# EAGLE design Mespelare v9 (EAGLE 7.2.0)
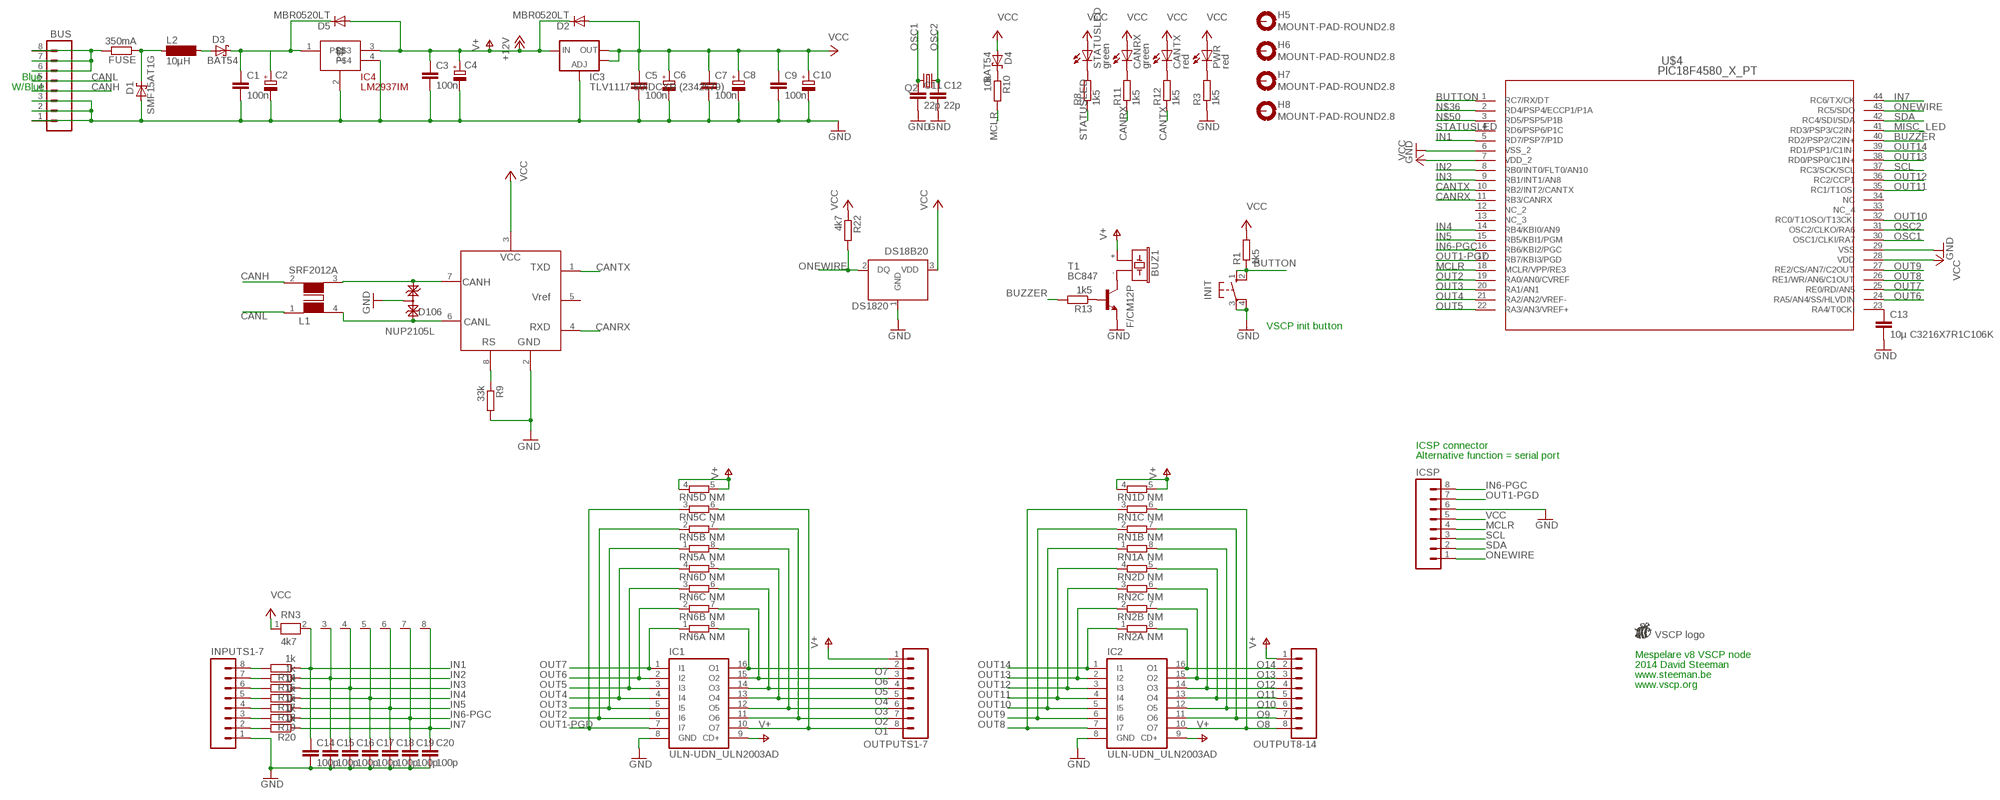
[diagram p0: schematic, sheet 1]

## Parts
BUS  M083.5MM-8  [SCREWTERMINAL-3.5MM-8]
BUZ1  F/CM12P  [F/CM12P]
C1  100n  C-EUC1206K  [C1206K]
C2  CPOL-EUC  [PANASONIC_C]
C3  100n  C-EUC1206K  [C1206K]
C4  CPOL-EUC  [PANASONIC_C]
C5  100n  C-EUC1206K  [C1206K]
C6  CPOL-EUC  [PANASONIC_C]
C7  100n  C-EUC1206K  [C1206K]
C8  CPOL-EUC  [PANASONIC_C]
C9  100n  C-EUC1206K  [C1206K]
C10  CPOL-EUC  [PANASONIC_C]
C11  22p  C-EUC1206  [C1206]
C12  22p  C-EUC1206  [C1206]
C13  10µ C3216X7R1C106K  C-EUC1206K  [C1206K]
C14  100p  C-EUC1206  [C1206]
C15  100p  C-EUC1206  [C1206]
C16  100p  C-EUC1206  [C1206]
C17  100p  C-EUC1206  [C1206]
C18  100p  C-EUC1206  [C1206]
C19  100p  C-EUC1206  [C1206]
C20  100p  C-EUC1206  [C1206]
CANRX  green  LEDCHIPLED_1206  [CHIPLED_1206]
CANTX  red  LEDCHIPLED_1206  [CHIPLED_1206]
D1  SMF15AT1G  SMF5.0AT1  [SOD123FL]
D2  MBR0520LT  [SOD123]
D3  BAT54  [SOT23]
D4  BAT54  [SOT23]
D5  MBR0520LT  [SOD123]
D106  NUP2105L  NUP2105LSOT23  [DIODE_SOT23]
DS18B20  DS1820  [TO-92]
FUSE  350mA  R-EU_M1206  [M1206]
H5  MOUNT-PAD-ROUND2.8  [2,2-PAD2]
H6  MOUNT-PAD-ROUND2.8  [2,2-PAD2]
H7  MOUNT-PAD-ROUND2.8  [2,2-PAD2]
H8  MOUNT-PAD-ROUND2.8  [2,2-PAD2]
IC1  ULN-UDN_ULN2003AD  [ULN-UDN_SO16]
IC2  ULN-UDN_ULN2003AD  [ULN-UDN_SO16]
IC3  TLV1117-50IDCYR (2342579)  LD117ASTR  [SOT223]
IC4  LM2937IM  [SOT223]
ICSP  M083.5MM-8  [SCREWTERMINAL-3.5MM-8]
INIT  10-XX  [B3F-10XX]
INPUTS1-7  M083.5MM-8  [SCREWTERMINAL-3.5MM-8]
L1  SRF2012A  [SRF2012A]
L2  10µH  SM-NE45  [SM-NE45]
OUTPUT8-14  M083.5MM-8  [SCREWTERMINAL-3.5MM-8]
OUTPUTS1-7  M083.5MM-8  [SCREWTERMINAL-3.5MM-8]
PWR  red  LEDCHIPLED_1206  [CHIPLED_1206]
Q2  CRYSTALHC49UP  [HC49UP]
R1  1k5  R-EU_M1206  [M1206]
R3  1k5  R-EU_M1206  [M1206]
R8  1k5  R-EU_M1206  [M1206]
R9  33k  R-EU_M1206  [M1206]
R10  10k  R-EU_M1206  [M1206]
R11  1k5  R-EU_M1206  [M1206]
R12  1k5  R-EU_M1206  [M1206]
R13  1k5  R-EU_M1206  [M1206]
R14  1k  R-EU_M1206  [M1206]
R15  1k  R-EU_M1206  [M1206]
R16  1k  R-EU_M1206  [M1206]
R17  1k  R-EU_M1206  [M1206]
R18  1k  R-EU_M1206  [M1206]
R19  1k  R-EU_M1206  [M1206]
R20  1k  R-EU_M1206  [M1206]
R22  4k7  R-EU_M1206  [M1206]
RN1  NM  4R-NEXBS8V  [EXBS8V]
RN2  NM  4R-NEXBS8V  [EXBS8V]
RN3  4k7  RN07  [RN-8]
RN5  NM  4R-NEXBS8V  [EXBS8V]
RN6  NM  4R-NEXBS8V  [EXBS8V]
STATUSLED  green  LEDCHIPLED_1206  [CHIPLED_1206]
T1  BC847  [SOT23]
U101  MCP2551  [MCP2551]
U$1  VSCP_LOGO2  [VSCP_LOGO2]
U$4  PIC18F4580_X_PT  [TQFP44_MC]

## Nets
BUTTON: INIT.1(S) INIT.2(S1) R1.1 U$4.1(RC7/RX/DT)
BUZZER: R13.2 U$4.40(RD2/PSP2/C2IN+)
CANH: BUS.4 L1.2
CANL: BUS.5 L1.1
CANRX: R11.1 U101.4(RXD) U$4.11(RB3/CANRX)
CANTX: R12.1 U101.1(TXD) U$4.10(RB2/INT2/CANTX)
GND: BUS.1 BUS.2 BUS.3 C1.2 C2.- C3.2 C4.- C5.2 C6.- C7.2 C8.- C9.2 C10.- C11.2 C12.2 C13.2 C14.2 C15.2 C16.2 C17.2 C18.2 C19.2 C20.2 D1.A D106.3(A) DS18B20.1(GND) IC1.8(GND) IC2.8(GND) IC3.1(ADJ) IC4.2 IC4.4 ICSP.6 INIT.3(P) INIT.4(P1) INPUTS1-7.1 R3.1 R9.2 T1.2(E) U101.2(GND) U$4.6(VSS_2) U$4.29(VSS)
I1: INPUTS1-7.8 R14.2
I2: INPUTS1-7.7 R15.2
I3: INPUTS1-7.6 R16.2
I4: INPUTS1-7.5 R17.2
I5: INPUTS1-7.4 R18.2
I6: INPUTS1-7.3 R19.2
I7: INPUTS1-7.2 R20.2
IN1: C14.1 R14.1 RN3.2 U$4.5(RD7/PSP7/P1D)
IN2: C15.1 R15.1 RN3.3 U$4.8(RB0/INT0/FLT0/AN10)
IN3: C16.1 R16.1 RN3.4 U$4.9(RB1/INT1/AN8)
IN4: C17.1 R17.1 RN3.5 U$4.14(RB4/KBI0/AN9)
IN5: C18.1 R18.1 RN3.6 U$4.15(RB5/KBI1/PGM)
IN6-PGC: C19.1 ICSP.8 R19.1 RN3.7 U$4.16(RB6/KBI2/PGC)
IN7: C20.1 R20.1 RN3.8 U$4.44(RC6/TX/CK)
MCLR: ICSP.4 R10.2 U$4.18(MCLR/VPP/RE3)
MISC_LED: U$4.41(RD3/PSP3/C2IN-)
N$1: D106.1(K1) L1.4 U101.6(CANL)
N$2: D106.2(K2) L1.3 U101.7(CANH)
N$3: C13.1 U$4.23(RA4/T0CKI)
N$5: C1.1 C2.+ D3.3(C) D5.C IC4.1
N$6: D1.C FUSE.1 L2.1
N$7: R9.1 U101.8(RS)
N$14: BUS.6 BUS.7 BUS.8 FUSE.2
N$15: D4.3(C) R10.1
N$16: R8.2 STATUSLED.C
N$19: D3.1(A) L2.2
N$20: BUZ1.- T1.3(C)
N$24: PWR.C R3.2
N$27: R13.1 T1.1(B)
N$36: U$4.2(RD4/PSP4/ECCP1/P1A)
N$50: U$4.3(RD5/PSP5/P1B)
N$53: CANRX.C R11.2
N$54: CANTX.C R12.2
O1: IC1.10(O7) OUTPUTS1-7.8 RN5.6
O2: IC1.11(O6) OUTPUTS1-7.7 RN5.7
O3: IC1.12(O5) OUTPUTS1-7.6 RN5.8
O4: IC1.13(O4) OUTPUTS1-7.5 RN6.5
O5: IC1.14(O3) OUTPUTS1-7.4 RN6.6
O6: IC1.15(O2) OUTPUTS1-7.3 RN6.7
O7: IC1.16(O1) OUTPUTS1-7.2 RN6.8
O8: IC2.10(O7) OUTPUT8-14.8 RN1.6
O9: IC2.11(O6) OUTPUT8-14.7 RN1.7
O10: IC2.12(O5) OUTPUT8-14.6 RN1.8
O11: IC2.13(O4) OUTPUT8-14.5 RN2.5
O12: IC2.14(O3) OUTPUT8-14.4 RN2.6
O13: IC2.15(O2) OUTPUT8-14.3 RN2.7
O14: IC2.16(O1) OUTPUT8-14.2 RN2.8
ONEWIRE: DS18B20.2(DQ) ICSP.1 R22.2 U$4.43(RC5/SDO)
OSC1: C11.1 Q2.2 U$4.30(OSC1/CLKI/RA7)
OSC2: C12.1 Q2.1 U$4.31(OSC2/CLKO/RA6)
OUT1-PGD: IC1.7(I7) ICSP.7 RN5.3 U$4.17(RB7/KBI3/PGD)
OUT2: IC1.6(I6) RN5.2 U$4.19(RA0/AN0/CVREF)
OUT3: IC1.5(I5) RN5.1 U$4.20(RA1/AN1)
OUT4: IC1.4(I4) RN6.4 U$4.21(RA2/AN2/VREF-)
OUT5: IC1.3(I3) RN6.3 U$4.22(RA3/AN3/VREF+)
OUT6: IC1.2(I2) RN6.2 U$4.24(RA5/AN4/SS/HLVDIN)
OUT7: IC1.1(I1) RN6.1 U$4.25(RE0/RD/AN5)
OUT8: IC2.7(I7) RN1.3 U$4.26(RE1/WR/AN6/C1OUT)
OUT9: IC2.6(I6) RN1.2 U$4.27(RE2/CS/AN7/C2OUT)
OUT10: IC2.5(I5) RN1.1 U$4.32(RC0/T1OSO/T13CKI)
OUT11: IC2.4(I4) RN2.4 U$4.35(RC1/T1OSI)
OUT12: IC2.3(I3) RN2.3 U$4.36(RC2/CCP1)
OUT13: IC2.2(I2) RN2.2 U$4.38(RD0/PSP0/C1IN+)
OUT14: IC2.1(I1) RN2.1 U$4.39(RD1/PSP1/C1IN-)
SCL: ICSP.3 U$4.37(RC3/SCK/SCL)
SDA: ICSP.2 U$4.42(RC4/SDI/SDA)
STATUSLED: R8.1 U$4.4(RD6/PSP6/P1C)
V+: BUZ1.+ C3.1 C4.+ D2.C D5.A IC1.9(CD+) IC2.9(CD+) IC3.3(IN) IC4.3 OUTPUT8-14.1 OUTPUTS1-7.1 RN1.4 RN1.5 RN5.4 RN5.5 ; supply symbol labelled +12V
VCC: C5.1 C6.+ C7.1 C8.+ C9.1 C10.+ CANRX.A CANTX.A D2.A D4.1(A) DS18B20.3(VDD) IC3.2(OUT1) IC3.4(OUT) ICSP.5 PWR.A R1.2 R22.1 RN3.1 STATUSLED.A U101.3(VCC) U$4.7(VDD_2) U$4.28(VDD)
Unconnected: H5.B2,8(MOUNT) H6.B2,8(MOUNT) H7.B2,8(MOUNT) H8.B2,8(MOUNT) U101.5(VREF) U$4.12(NC_2) U$4.13(NC_3) U$4.33(NC_4) U$4.34(NC)

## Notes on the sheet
- Blue
- W/Blue
- VSCP init button
- ICSP connector
- Alternative function = serial port
- Mespelare v8 VSCP node
- 2014 David Steeman
- www.steeman.be
- www.vscp.org

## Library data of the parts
BUS ICSP INPUTS1-7 OUTPUT8-14 OUTPUTS1-7 = SparkFun-Connectors:M08: Header 8 Standard 8-pin 0.1" header. Use with straight break away headers (SKU : PRT-00116), right angle break away headers (PRT-00553), swiss pins (PRT-00743), machine pins (PRT-00117), and female headers (PRT-00115).
BUZ1 = buzzer:F/CM12P: BUZZER
C1 C3 C5 C7 C9 C11-C20 = rcl:C-EU: CAPACITOR, European symbol
C2 C4 C6 C8 C10 = rcl:CPOL-EU: POLARIZED CAPACITOR, European symbol
CANRX CANTX PWR STATUSLED = led:LED: LED
D1 = diode:SMF5.0AT1: 200 W Transient Voltage Suppressor
D2 D5 = diode:MBR0520LT: SCHOTTKY BARRIER RECTIFIER
D3 D4 = diode:BAT54: Schottky Diodes
D106 = Hasselt_v20:NUP2105L: Dual DIODE Cathode-Anode|Anode-Cathode
DS18B20 = DS1820:DS1820: DS1820 - 1-Wire Digital Thermometer
FUSE R1 R3 R8-R20 R22 = rcl:R-EU_: RESISTOR, European symbol
H5-H8 = holes:MOUNT-PAD-ROUND: MOUNTING PAD, round
IC1 IC2 = Hasselt_v20:ULN-UDN_ULN2003A: DRIVER ARRAY
IC3 = v-reg:LD117A?*: Low drop fixed and adjustable positive voltage regulators 1 A Source: http://www.st.com/stonline/products/literature/ds/7194/ld1117axx.pdf
IC4 = v-reg:LM2937IM
INIT = switch-omron:10-XX: OMRON SWITCH
L1 = Hasselt_v20:SRF2012A
L2 = inductor-neosid:SM-NE45: INDUCTOR; OC_FARNELL: unknown; OC_NEWARK: unknown
Q2 = crystal:CRYSTAL: CRYSTAL
RN1 RN2 RN5 RN6 = resistor-dil:4R-N: Array Chip Resistor Source: RS Component / Phycomp
RN3 = resistor-net:RN07: RESISTOR NETWORK; OC_FARNELL: unknown; OC_NEWARK: unknown
T1 = transistor:BC847: NPN TRANSISTOR
U101 = Hasselt_v20:MCP2551
U$1 = VSCP_logo:VSCP_LOGO2
U$4 = PIC18F4580 exported:PIC18F4580_X_PT

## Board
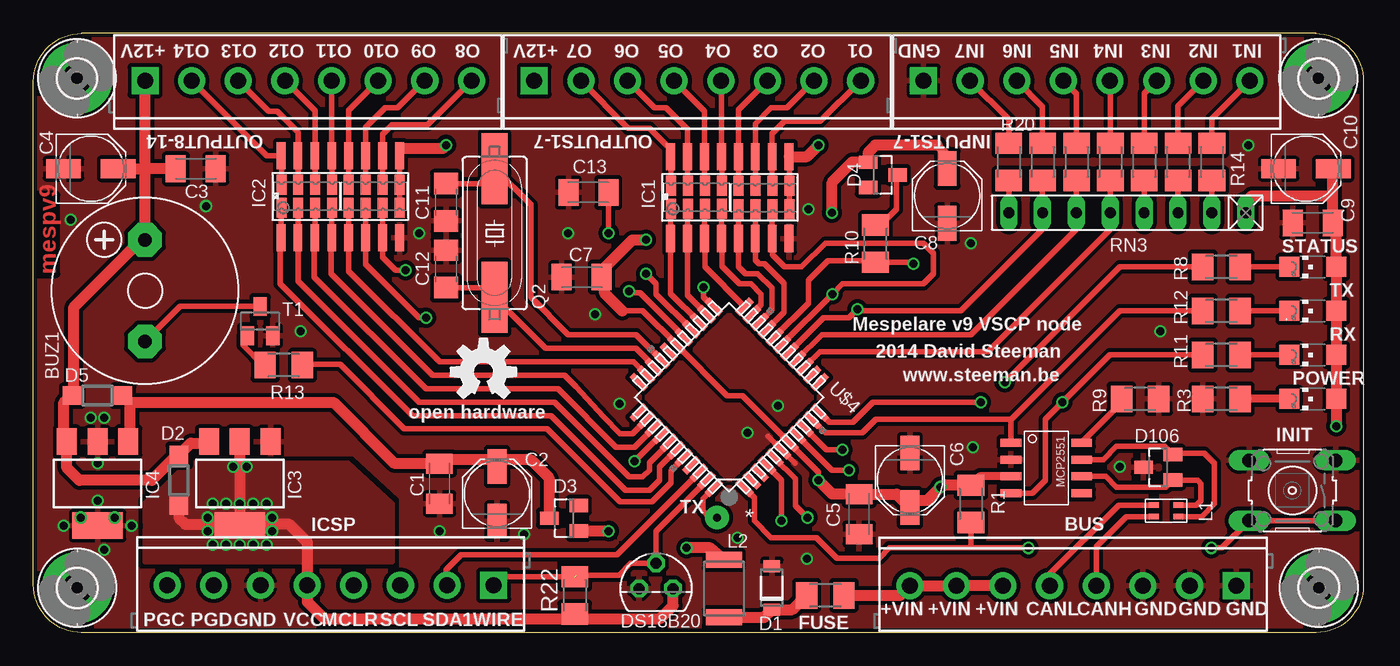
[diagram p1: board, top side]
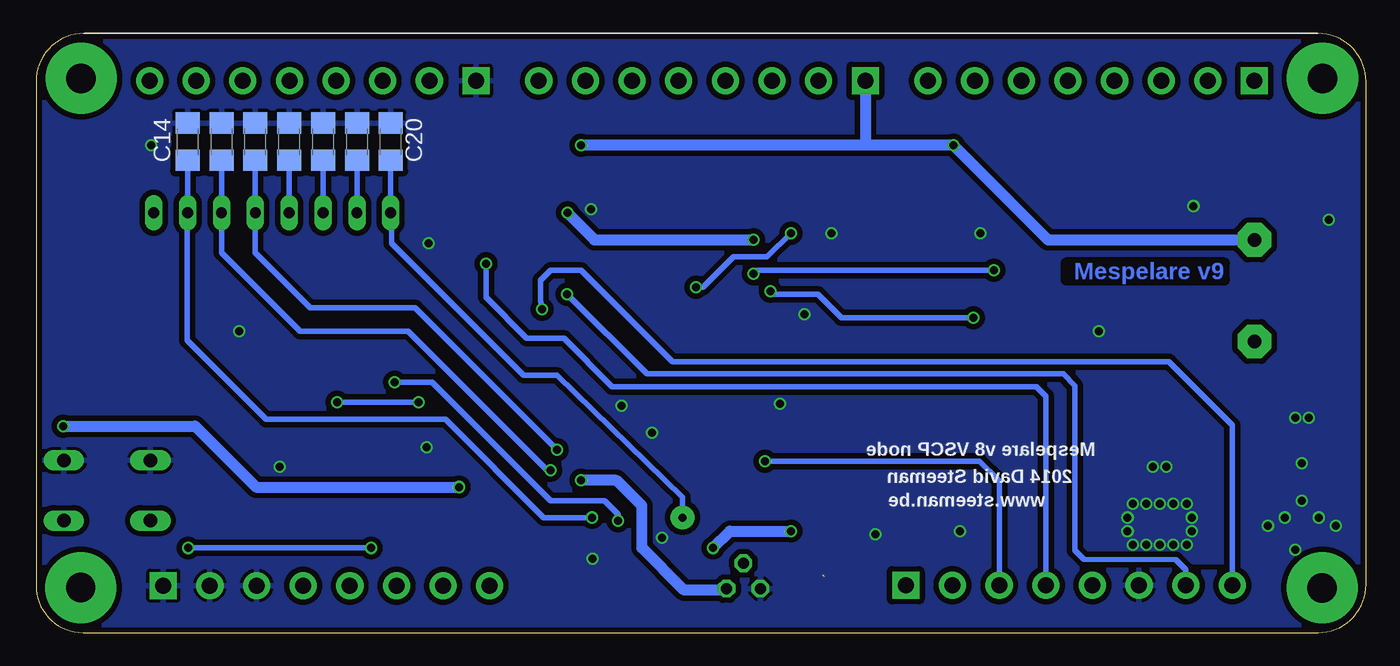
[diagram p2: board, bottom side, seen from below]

Size 99.82 x 44.96 mm. Coordinates in mm from the lower left corner, seen from the top.
Outline: 3.64,44.96 arc90 0,41.32 0,3.61 arc90 3.61,0 96.29,0 arc90 99.82,3.53 99.82,41.35 arc90 96.21,44.96
Outline: 96.29,44.96 3.61,44.96
Copper layers (1*16): Top 0.035mm / dielectric 1.5mm / Bottom 0.035mm
Design rules "SeeedStudio_2layer_DRU_no_angle_20140221": minimum track width 6mil, minimum drill 12mil, track to track 6mil, track to pad 6mil, pad to pad 6mil, via to via 6mil, smd to smd 0mil, copper to edge 10mil, drill to drill 10mil, minimum pad ring 10mil, minimum via ring 6mil, stop-mask expansion 2mil, vias tented up to drill 100mil, thermal gap 10mil
tRestrict: area 18.5,32.5 to 26.7,33; area 47.5,32.5 to 55.9,33; area 72.4,36.3 to 89.2,37.1
bRestrict: area 72.4,36.3 to 89.2,37.1

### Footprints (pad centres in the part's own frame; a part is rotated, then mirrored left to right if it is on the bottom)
SCREWTERMINAL-3.5MM-8 = drill 1.2 pad 2.032 square: 1 0,0 | drill 1.2 pad 2.032: 2 3.5,0; 3 7,0; 4 10.5,0; 5 14,0; 6 17.5,0; 7 21,0; 8 24.5,0
F/CM12P = drill 1.016 pad 2.54 octagon: + 3.81,0; - -3.81,0
C1206K = smd 1.5 x 2: 1 -1.5,0; 2 1.5,0
PANASONIC_C = smd 2.6 x 1.4: + 2.05,0; - -2.05,0
C1206 = smd 1.6 x 1.8: 1 -1.4,0; 2 1.4,0
CHIPLED_1206 = smd 1.5 x 1.5: A 0,-1.75; C 0,1.75
SOD123FL = smd 0.91 x 1.22: A 1.625,0; C -1.625,0
SOD123 = smd 1.4 x 1.4: A 1.9,0; C -1.9,0
SOT23 = smd 1 x 1.4: 1 -0.95,-1.1; 2 0.95,-1.1; 3 0,1.1
DIODE_SOT23 = smd 1 x 1.4: 1 -0.95,-1.1; 2 0.95,-1.1; 3 0,1.1
TO-92 = drill 0.813 pad 1.27 octagon: 1 -1.27,0; 2 0,1.905; 3 1.27,0
M1206 = smd 1.6 x 2: 1 -1.4,0; 2 1.4,0
2,2-PAD2 = drill 2.2 pad 5.334: B2,8 0,0
ULN-UDN_SO16 = smd 0.66 x 2.032: 1 -4.445,-3.073; 2 -3.175,-3.073; 3 -1.905,-3.073; 4 -0.635,-3.073; 5 0.635,-3.073; 6 1.905,-3.073; 7 3.175,-3.073; 8 4.445,-3.073; 9 4.445,3.073; 10 3.175,3.073; 11 1.905,3.073; 12 0.635,3.073; 13 -0.635,3.073; 14 -1.905,3.073; 15 -3.175,3.073; 16 -4.445,3.073
SOT223 = smd 1.5 x 2: 1 -2.3,-3.15; 2 0,-3.15; 3 2.3,-3.15 | smd 3.8 x 2: 4 0,3.15
B3F-10XX = drill 1.016 long: 1 -3.251,2.261; 2 3.251,2.261; 3 -3.251,-2.261; 4 3.251,-2.261
SRF2012A = smd 0.4 x 0.75: 1 -0.068,-0.432; 2 -0.932,-0.432; 3 -0.932,-2.294; 4 -0.068,-2.294
SM-NE45 = smd 1.2 x 2.7: 1 -2.15,0; 2 2.15,0
HC49UP = smd 5.334 x 1.93: 1 -4.826,0; 2 4.826,0
EXBS8V = smd 0.75 x 1.5: 1 -1.905,-0.87; 2 -0.635,-0.87; 3 0.635,-0.87; 4 1.905,-0.87; 5 1.905,0.87; 6 0.635,0.87; 7 -0.635,0.87; 8 -1.905,0.87
RN-8 = drill 0.813 long: 1 -8.89,0; 2 -6.35,0; 3 -3.81,0; 4 -1.27,0; 5 1.27,0; 6 3.81,0; 7 6.35,0; 8 8.89,0
MCP2551 = smd 0.6 x 1.55: 1 -1.905,-2.65; 2 -0.635,-2.65; 3 0.635,-2.65; 4 1.905,-2.65; 5 1.905,2.65; 6 0.635,2.65; 7 -0.635,2.65; 8 -1.905,2.65
TQFP44_MC = smd 1.473 x 0.508: 1 -5.613,3.988; 2 -5.613,3.2; 3 -5.613,2.388; 4 -5.613,1.6; 5 -5.613,0.787; 6 -5.613,0; 7 -5.613,-0.787; 8 -5.613,-1.6; 9 -5.613,-2.388; 10 -5.613,-3.2; 11 -5.613,-3.988; 23 5.613,-3.988; 24 5.613,-3.2; 25 5.613,-2.388; 26 5.613,-1.6; 27 5.613,-0.787; 28 5.613,0; 29 5.613,0.787; 30 5.613,1.6; 31 5.613,2.388; 32 5.613,3.2; 33 5.613,3.988 | smd 0.508 x 1.473: 12 -3.988,-5.613; 13 -3.2,-5.613; 14 -2.388,-5.613; 15 -1.6,-5.613; 16 -0.787,-5.613; 17 0,-5.613; 18 0.787,-5.613; 19 1.6,-5.613; 20 2.388,-5.613; 21 3.2,-5.613; 22 3.988,-5.613; 34 3.988,5.613; 35 3.2,5.613; 36 2.388,5.613; 37 1.6,5.613; 38 0.787,5.613; 39 0,5.613; 40 -0.787,5.613; 41 -1.6,5.613; 42 -2.388,5.613; 43 -3.2,5.613; 44 -3.988,5.613

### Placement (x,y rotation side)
BUS  90.27,3.53 180 top
BUZ1  8.38,25.65 90 top
C1  30.48,11.18 270 top
C2  34.8,10.41 90 top
C3  12.19,34.8 0 top
C4  4.32,34.8 0 top
C5  61.98,8.89 270 top
C6  65.79,11.43 270 top
C7  41.15,26.67 180 top
C8  68.58,32.77 90 top
C9  96.01,30.73 180 top
C10  95.5,34.8 0 top
C11  30.96,32.28 270 top
C12  30.96,27.28 90 top
C13  41.66,33.02 180 top
C14  88.44,36.83 90 bottom
C15  85.9,36.83 90 bottom
C16  83.36,36.83 90 bottom
C17  80.82,36.83 90 bottom
C18  78.28,36.83 90 bottom
C19  75.74,36.83 90 bottom
C20  73.2,36.83 90 bottom
CANRX  96.01,20.83 90 top
CANTX  96.01,24.13 90 top
D1  55.42,3.35 90 top
D2  10.92,11.43 270 top
D3  39.83,8.59 90 top
D4  63.75,34.34 270 top
D5  4.83,17.78 180 top
D106  84.42,12.4 90 top
DS18B20  46.74,3.3 0 top
FUSE  59.44,2.79 0 top
H5  3.3,3.35 0 top
H6  3.28,41.58 0 top
H7  96.47,3.38 0 top
H8  96.44,41.58 0 top
IC1  52.27,32.64 0 top
IC2  23.04,32.7 0 top
IC3  15.49,11.18 180 top
IC4  4.83,11.18 180 top
ICSP  34.54,3.56 180 top
INIT  94.49,10.67 180 top
INPUTS1-7  66.8,41.4 0 top
L1  83.65,9.63 90 top
L2  51.82,3.3 90 top
OUTPUT8-14  8.38,41.4 0 top
OUTPUTS1-7  37.59,41.4 0 top
PWR  96.01,17.53 90 top
Q2  34.62,29.97 90 top
R1  70.36,9.65 90 top
R3  89.15,17.53 0 top
R8  89.15,27.43 0 top
R9  83.06,17.53 0 top
R10  63.2,29.18 270 top
R11  89.15,20.83 0 top
R12  89.15,24.13 0 top
R13  18.8,20.07 0 top
R14  88.44,35.31 90 top
R15  85.9,35.31 90 top
R16  83.36,35.31 90 top
R17  80.82,35.31 90 top
R18  78.28,35.31 90 top
R19  75.74,35.31 90 top
R20  73.2,35.31 90 top
R22  40.64,2.79 90 top
RN1  25.59,32.73 0 top
RN2  20.53,32.73 0 top
RN3  82.09,31.5 180 top
RN5  54.84,32.64 0 top
RN6  49.76,32.66 0 top
STATUSLED  96.01,27.43 90 top
T1  17.02,23.37 0 top
U101  76.02,12.35 270 top
U$1  69.34,24.38 0 top
U$3  [OSHW-LOGO-M]  33.78,19.56 0 top
U$4  52.22,17.65 135 top

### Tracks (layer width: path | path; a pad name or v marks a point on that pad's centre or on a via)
BUTTON  (via drill 0.6)
  Top 0.406: INIT.1 INIT.2 | INIT.2 90.45,8.41 | U$4.1 54.1,10.13 54.1,8.38 55.37,7.11 58.78,7.11 60.3,5.59 63.5,5.59 64.26,6.35 70.36,6.35 | 70.36,6.35 v74.68,6.35 | R1.1 70.36,6.35 | v88.39,6.35 89.18,6.35 INIT.2
  Bottom 0.406: v74.68,6.35 v88.39,6.35
BUZZER
  Top 0.406: U$4.40 48.81,13.1 47.85,12.14 47.85,11.23 46.43,9.8 44.04,9.8 38.56,15.29 27.84,15.29 23.01,20.12 20.2,20.12 R13.2
CANH
  Top 0.406: L1.2 82.04,8.7 79.79,6.44 79.77,6.44 BUS.4
CANL
  Top 0.406: L1.1 81.44,9.56 76.29,4.4 76.27,4.4 BUS.5
CANRX  (via drill 0.6)
  Top 0.406: v71.12,17.27 62.99,17.27 61.52,15.8 59.74,15.8 59.04,16.5 U$4.11 | R11.1 87.75,20.85 80.8,20.85 v77.22,17.27 75.95,16 75.95,11.43 74.96,10.45 U101.4
  Bottom 0.406: v71.12,17.27 v77.22,17.27
CANTX
  Top 0.406: 73.37,15.96 81.53,24.13 R12.1 | U$4.10 58.48,15.95 59.44,14.99 62.23,14.99 63.25,16 73.33,16 73.37,15.96 | U101.1 73.37,15.96
GND  (via drill 0.6)
  Top 0.406: U$4.6 56.19,13.66 | 56.19,13.66 57.15,12.7 | 56.19,13.66 55.12,14.73
  other vias: 53.59,14.99 12.95,32 81.53,12.45 52.83,7.11 70.51,13.92 43.99,17.17 91.19,36.58 28.96,29.97 2.79,30.99 42.16,23.88 84.58,22.61 58.17,31.75 70.36,29.21 58.06,5.54 30.48,7.62 36.83,7.37 55.88,17.02 20.07,22.61 4.83,9.91 7.37,8 5.33,6.22 2.29,8 4.32,16.13 4.83,12.7 3.56,8.64 6.1,8.64 5.33,16.13 40.13,29.97
  pour Top (isolate 0.305, rank 6): 0,0 99.82,0 99.57,44.7 0,44.7
  pour Bottom (isolate 0.406, rank 6): 0,0 99.82,0 99.82,44.96 0,44.96
I1
  Top 0.406: R14.2 88.44,38.54 INPUTS1-7.8
I2
  Top 0.406: R15.2 85.9,39.5 INPUTS1-7.7
I3
  Top 0.406: R16.2 83.36,40.46 INPUTS1-7.6
I4
  Top 0.406: R17.2 80.82,41.38 INPUTS1-7.5
I5
  Top 0.406: R18.2 78.28,40.42 INPUTS1-7.4
I6
  Top 0.406: R19.2 75.74,39.46 INPUTS1-7.3
I7
  Top 0.406: R20.2 73.2,38.5 INPUTS1-7.2
IN1  (via drill 0.6)
  Top 0.406: R14.1 RN3.2 | U$4.5 55.64,13.1 57.2,11.53 57.2,9.53 v58.09,8.64
  Bottom 0.406: C14.1 RN3.2 88.14,31.95 88.39,32.26 88.49,31.9 88.49,21.95 82.55,16 69.09,16 61.72,8.64 v58.09,8.64
IN2  (via drill 0.6)
  Top 0.406: R15.1 RN3.3 | U$4.8 59.94,12.19 v61.22,12.19
  Bottom 0.406: C15.1 RN3.3 85.9,28.5 80.01,22.61 71.88,22.61 61.47,12.19 v61.22,12.19
IN3  (via drill 0.6)
  Top 0.406: R16.1 RN3.4 | v60.71,13.72 59.54,13.72 U$4.9
  Bottom 0.406: C16.1 RN3.4 83.36,28.5 79.25,24.38 71.37,24.38 v60.71,13.72
IN4
  Top 0.406: R17.1 RN3.5 80.82,30.28 71.63,21.08 59.03,21.08 U$4.14
  Bottom 0.406: C17.1 RN3.5
IN5
  Top 0.406: R18.1 RN3.6 78.28,30.28 70.36,22.35 59.18,22.35 U$4.15
  Bottom 0.406: C18.1 RN3.6
IN6-PGC  (via drill 0.6)
  Top 0.406: R19.1 RN3.7 75.74,30.28 69.6,24.13 61.72,24.13 | 61.72,24.13 61.21,23.62 59.3,23.62 U$4.16 | 61.72,24.13 v61.85,24.26
  Bottom 0.406: C19.1 RN3.7 75.77,31.42 | v61.85,24.26 61.98,24.89 61.98,26.42 61.21,27.18 58.93,27.18 52.07,20.32 14.8,20.32 10.04,15.57 ICSP.8
IN7  (via drill 0.6 pad 1.78)
  Top 0.406: RN3.8 R20.1 | U$4.44 51.05,10.86 50.24,10.06 50.24,9.14 50.75,8.64 v51.31,8.64
  Bottom 0.406: C20.1 RN3.8 73.15,32.21 73.15,29.21 63.25,19.3 60.71,19.3 51.31,10.16 v51.31,8.64
MCLR  (via drill 0.6)
  Top 0.406: 55.64,22.21 U$4.18 58.17,24.71 58.17,26.42 59.64,27.89 62.54,27.89 R10.2 65.94,27.79 v66.04,27.69
  Bottom 0.406: v66.04,27.69 66.04,25.15 62.99,22.1 60.2,22.1 56.59,18.44 24.76,18.44 24.04,17.72 ICSP.4
N$1
  Top 0.406: U101.6 80.49,11.72 81.28,10.92 84.99,10.92 D106.1 86.05,11.43 87.38,11.43 87.63,11.18 87.63,9.91 87.29,9.56 L1.4
N$2
  Top 0.406: U101.7 80.3,12.99 81.28,13.97 84.9,13.97 D106.2 86.14,13.46 87.88,13.46 88.65,12.7 88.65,9.65 87.69,8.7 L1.3
N$3  (via drill 0.6)
  Top 0.406: U$4.23 51,24.44 50.29,25.15 v50.29,25.91 | v43.18,29.97 43.18,33.02 C13.1
  Bottom 0.406: v50.29,25.91 49.78,25.91 47.5,28.19 44.96,28.19 v43.18,29.97
N$5
  Top 0.61: 34.82,12.95 C2.+ | 30.69,12.97 C1.1
  Top 0.813: D3.3 38.73,11.57 37.34,12.95 34.82,12.95 | C2.+ 34.8,12.95 30.69,12.97 | 7.29,17.27 22.53,17.27 27.12,12.68 C1.1 | 7.29,17.27 D5.C | IC4.1 7.29,14.33 7.29,17.27
N$6
  Top 0.813: L2.1 54.85,1.15 D1.C 56.97,1.73 FUSE.1
N$7
  Top 0.406: R9.1 81.66,17.25 U101.8
N$14
  Top 0.813: BUS.6 BUS.7 BUS.8 65.03,2.79 FUSE.2
N$15
  Top 0.406: R10.1 64.11,31.09 64.77,31.75 64.77,34.41 D4.3
N$16
  Top 0.406: R8.2 STATUSLED.C
N$19  (via drill 0.6)
  Top 0.61: 40.94,7.62 D3.1
  Top 0.813: v43.18,7.62 40.94,7.62 | L2.2 50.8,6.35 v49.02,6.35
  Bottom 0.813: v49.02,6.35 47.75,7.62 v43.18,7.62
N$20
  Top 0.406: T1.3 11.01,24.47 BUZ1.-
N$24
  Top 0.61: PWR.C R3.2
N$27
  Top 0.406: T1.1 15.75,22.27 15.75,21.55 17.23,20.07 R13.1
N$53
  Top 0.406: R11.2 CANRX.C
N$54
  Top 0.406: R12.2 CANTX.C
O1
  Top 0.406: OUTPUTS1-7.8 59.04,38.35 56.39,38.35 55.45,37.41 IC1.10 55.45,33.73 RN5.6
O2
  Top 0.406: OUTPUTS1-7.7 56.56,39.37 55.37,39.37 54.18,38.18 IC1.11 54.18,33.73 RN5.7
O3
  Top 0.406: OUTPUTS1-7.6 52.91,39.22 IC1.12 52.91,33.73 RN5.8
O4
  Top 0.406: RN6.5 51.66,35.71 IC1.13 51.64,41.36 OUTPUTS1-7.5
O5
  Top 0.406: OUTPUTS1-7.4 50.37,39.13 IC1.14 50.37,33.76 RN6.6
O6
  Top 0.406: OUTPUTS1-7.3 46.62,39.37 47.5,39.37 49.1,37.77 IC1.15 49.1,33.76 RN6.7
O7
  Top 0.406: RN6.8 47.85,35.71 IC1.16 47.83,36.25 46.23,37.85 44.65,37.85 OUTPUTS1-7.2
O8
  Top 0.406: RN1.6 26.21,33.8 IC2.10 26.21,37.39 26.92,38.1 29.58,38.1 OUTPUT8-14.8
O9
  Top 0.406: RN1.7 24.94,33.8 IC2.11 24.94,37.9 26.42,39.37 27.35,39.37 OUTPUT8-14.7
O10
  Top 0.406: RN1.8 23.67,33.8 IC2.12 23.67,39.19 OUTPUT8-14.6
O11
  Top 0.406: RN2.5 22.43,35.75 IC2.13 22.4,41.38 OUTPUT8-14.5 22.35,41.43
O12
  Top 0.406: RN2.6 21.13,33.8 IC2.14 21.13,39.15 OUTPUT8-14.4
O13
  Top 0.406: RN2.7 19.86,33.8 IC2.15 19.86,37.54 18.29,39.12 17.67,39.12 OUTPUT8-14.3
O14
  Top 0.406: RN2.8 18.62,35.78 IC2.16 17.51,35.78 OUTPUT8-14.2
ONEWIRE  (1 unrouted)
  Top 0.406: U$4.43 50.52,11.4 46.74,7.62 DS18B20.2 44.83,5.21 43.94,4.32 40.76,4.32 | ICSP.1 35.18,4.19 R22.2
OSC1
  Top 0.406: U$4.30 47.07,20.49 45.21,22.35 40.13,22.35 37.34,25.15 37.34,32.08 Q2.2 33.51,33.68 C11.1
OSC2
  Top 0.406: U$4.31 46.57,19.98 45.21,21.34 38.43,21.34 Q2.1 33.89,25.88 C12.1
OUT1-PGD  (via drill 0.6)
  Top 0.406: RN5.3 55.45,31.57 IC1.7 55.47,29.57 55.47,28.35 56.39,27.43 57.66,27.43 59.44,29.21 66.8,29.21 67.56,28.45 67.56,26.92 66.8,26.16 60.73,26.16 v59.96,25.39 U$4.17
  Bottom 0.406: v59.96,25.39 53.98,19.41 22.72,19.41 21.84,18.53 21.84,6.19 21.18,5.52 14.29,5.46 13.54,4.72 ICSP.7
OUT2
  Top 0.406: RN5.2 54.18,31.57 IC1.6 54.2,29.54 54.2,27.94 54.46,27.69 54.86,27.69 56.34,26.21 56.34,24.03 U$4.19
OUT3
  Top 0.406: RN5.1 52.91,31.57 IC1.5 52.93,29.54 52.93,27.43 53.44,26.92 54.36,26.92 55.42,25.86 55.42,24.23 U$4.20
OUT4
  Top 0.406: RN6.4 51.64,31.59 IC1.4 | U$4.21 53.93,23.91 54.61,24.59 54.61,25.4 53.85,26.16 52.98,26.16 51.66,27.48 51.66,29.54 IC1.4 | 51.56,29.49 IC1.4
OUT5
  Top 0.406: RN6.3 50.37,31.59 IC1.3 50.39,29.54 50.39,27.43 U$4.22
OUT6
  Top 0.406: RN6.2 49.1,31.59 IC1.2 49.1,25.3 U$4.24
OUT7
  Top 0.406: RN6.1 47.83,31.59 IC1.1 47.83,25.42 U$4.25
OUT8  (via drill 0.6)
  Top 0.406: RN1.3 26.21,31.66 IC2.7 26.21,28.14 27.18,27.18 v27.94,27.18 | v45.98,26.92 46.74,26.16 46.74,25.4 U$4.26
  Bottom 0.406: v27.94,27.18 45.72,27.18 v45.97,26.92 v45.98,26.92
OUT9  (via drill 0.6)
  Top 0.406: RN1.2 24.94,31.66 IC2.6 24.94,27.64 28.96,23.62 v29.46,23.62 | U$4.27 48.79,22.18 48.79,22.23 45.52,25.5 44.7,25.5 v44.7,25.6
  Bottom 0.406: v29.46,23.62 39.37,23.62 41.15,25.4 44.57,25.4 44.7,25.53 v44.7,25.6
OUT10
  Top 0.406: RN1.1 23.67,31.66 IC2.5 23.67,27.13 30.48,20.32 45.03,20.32 U$4.32
OUT11
  Top 0.406: RN2.4 22.4,31.66 IC2.4 22.35,29.58 22.35,26.92 29.97,19.3 39.88,19.3 40.74,18.44 42.77,16.2 44.04,14.94 44.96,14.94 45.97,15.95 U$4.35
OUT12
  Top 0.406: RN2.3 21.13,31.66 IC2.3 21.08,29.58 21.08,26.67 29.46,18.29 39.37,18.29 43.74,13.92 45.11,13.92 U$4.36
OUT13
  Top 0.406: RN2.2 19.86,31.66 IC2.2 19.86,26.36 28.96,17.27 39.12,17.27 44.7,11.68 45.72,11.68 46.23,12.19 46.23,12.75 47.7,14.22 U$4.38
OUT14
  Top 0.406: RN2.1 18.59,31.66 IC2.1 18.54,29.58 18.54,26.16 28.45,16.26 38.86,16.26 44.45,10.67 46.23,10.67 46.99,11.43 46.99,12.45 48.23,13.68 U$4.39
SCL  (via drill 0.6)
  Top 0.406: U$4.37 47.07,14.82 v45.11,12.85
  Bottom 0.406: v45.11,12.85 29.02,12.85 27.54,11.38 ICSP.3
SDA
  Top 0.406: U$4.42 | ICSP.2 30.99,3.61 30.99,4.73 32.12,5.86 43.82,5.86 43.84,5.89 U$4.42 | 49.99,12 U$4.42
STATUSLED  (via drill 0.6)
  Top 0.406: R8.1 81.53,27.43 v72.9,18.8 | U$4.4 55.06,12.5 56.13,11.43 v56.13,8.38
  Bottom 0.406: v72.9,18.8 70.1,18.8 61.21,9.91 57.15,9.91 56.13,8.89 v56.13,8.38
V+  (via drill 0.6)
  Top 0.406: RN1.5 27.48,33.8 | RN1.4 RN1.5 | IC1.9 56.74,35.71 RN5.5 RN5.4 | IC2.9 27.48,33.8 RN1.5
  Top 0.61: 8.38,41.66 OUTPUT8-14.1 | IC2.9 27.48,36.12 27.69,36.32 | 30.72,36.32 30.72,36.33 30.74,36.33 v30.99,36.58
  Top 0.813: 27.69,36.32 30.72,36.32 | 8.38,34.8 BUZ1.+ 8.09,29.46 3.05,24.42 3.05,17.53 D5.A 2.29,17.27 2.29,14.33 IC4.3 2.53,12.36 3.45,11.43 8.89,11.43 10.79,13.33 D2.C 11.82,14.22 13.19,14.22 IC3.3 | 8.38,34.8 OUTPUT8-14.1 | IC1.9 58.06,35.71 v58.93,36.58 | C4.+ 8.38,34.8 | C3.1 8.38,34.8
  Bottom 0.61: 58.87,36.58 58.93,36.52 v58.93,36.58
  Bottom 0.813: BUZ1.+ 23.88,29.46 v30.99,36.58 37.59,36.58 | 37.59,36.58 58.87,36.58 v58.93,36.58 | OUTPUTS1-7.1 37.59,36.58
VCC  (via drill 0.6)
  Top 0.406: 97.79,26.7 STATUSLED.A | v58.93,11.43 58.93,12.04 56.75,14.22 U$4.7 53.21,17.78 52.07,17.78 48.25,21.6 U$4.28 45.76,24.12 45.72,24.13 44.2,24.13 | 40.64,1.27 R22.1 40.64,1.02 41.02,1.02
  Top 0.61: PWR.A 97.79,17.78 | 40.64,1.27 40.39,1.02 | 97.51,34.76 C10.+ | 97.79,30.2 C9.1 | 62.52,35.31 D4.1 62.64,35.46 | C8.+ 68.58,35.81 67.82,36.58 | 42.88,27.38 42.88,26.64 C7.1 | U101.3 71.02,11.72 R1.2
  Top 0.813: STATUSLED.A CANTX.A CANRX.A PWR.A | 97.79,26.7 97.79,30.2 | 97.79,17.78 v97.79,15.49 | 41.02,1.02 46.99,1.02 48.01,2.03 DS18B20.3 | 40.39,1.02 21.84,1.02 20.57,2.29 20.57,3.02 ICSP.5 20.57,3.56 20.57,6.76 19.21,8.13 15.49,8.13 | 44.2,24.13 42.88,25.45 42.88,26.64 | C9.1 97.51,32.77 | 97.51,32.77 97.51,34.76 | RN3.1 90.98,32.31 91.44,32.77 97.51,32.77 | v59.94,31.5 59.94,33.78 61.47,35.31 62.52,35.31 | 67.82,36.58 63.2,36.58 62.64,36.02 62.64,35.46 | 42.88,27.38 44.96,29.46 v45.97,29.46 | v58.93,11.43 59.97,10.39 C5.1 64.78,10.39 C6.+ 65.8,9.4 65.79,9.65 65.79,9.91 67.06,9.91 v68.07,10.92 68.2,11.05 R1.2 | D2.A 10.92,8.64 11.43,8.13 15.49,8.13 | 15.49,8.13 IC3.4 IC3.2
  Bottom 0.61: DS18B20.3 48.01,3.18
  Bottom 0.813: v58.93,11.43 56.26,11.43 54.36,9.53 54.36,6.35 51.19,3.18 48.01,3.18 | v97.79,15.49 87.88,15.49 83.31,10.92 v68.07,10.92 | v59.94,31.5 57.91,29.46 v45.97,29.46
  other vias: 13.08,8.64 14.48,9.65 15.49,9.65 16.51,9.65 13.46,9.65 13.46,6.6 13.08,7.62 16.51,6.6 17.53,6.6 17.91,7.62 14.99,12.45 16,12.45 17.91,8.64 15.49,6.6 14.48,6.6 17.53,9.65
  pour Top (isolate 0.406, no thermals): 8.38,5.33 8.38,9.65 11.43,12.7 23.62,12.7 26.92,9.65 26.92,5.33
  pour Bottom (isolate 0.406): 10.41,5.33 10.41,15.73 14.75,20.07 21.84,20.07 21.84,5.33

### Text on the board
Top: mespv9
Bottom: Mespelare v9
tPlace: +12V | O14 | O13 | O12 | O11 | O10 | O9 | O8 | +12V | O7 | O6 | O5 | O4 | O3 | O2 | O1 | GND | IN7 | IN6 | IN5 | IN4 | IN3 | IN2 | IN1 | STATUS | TX | Mespelare v9 VSCP node | RX | 2014 David Steeman | www.steeman.be | POWER | open hardware | TX | PGC | PGD | GND | VCC | MCLR | SCL | SDA | 1WIRE | +VIN | +VIN | +VIN | CANL | CANH | GND | GND | GND
bPlace: Mespelare v8 VSCP node | 2014 David Steeman | www.steeman.be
